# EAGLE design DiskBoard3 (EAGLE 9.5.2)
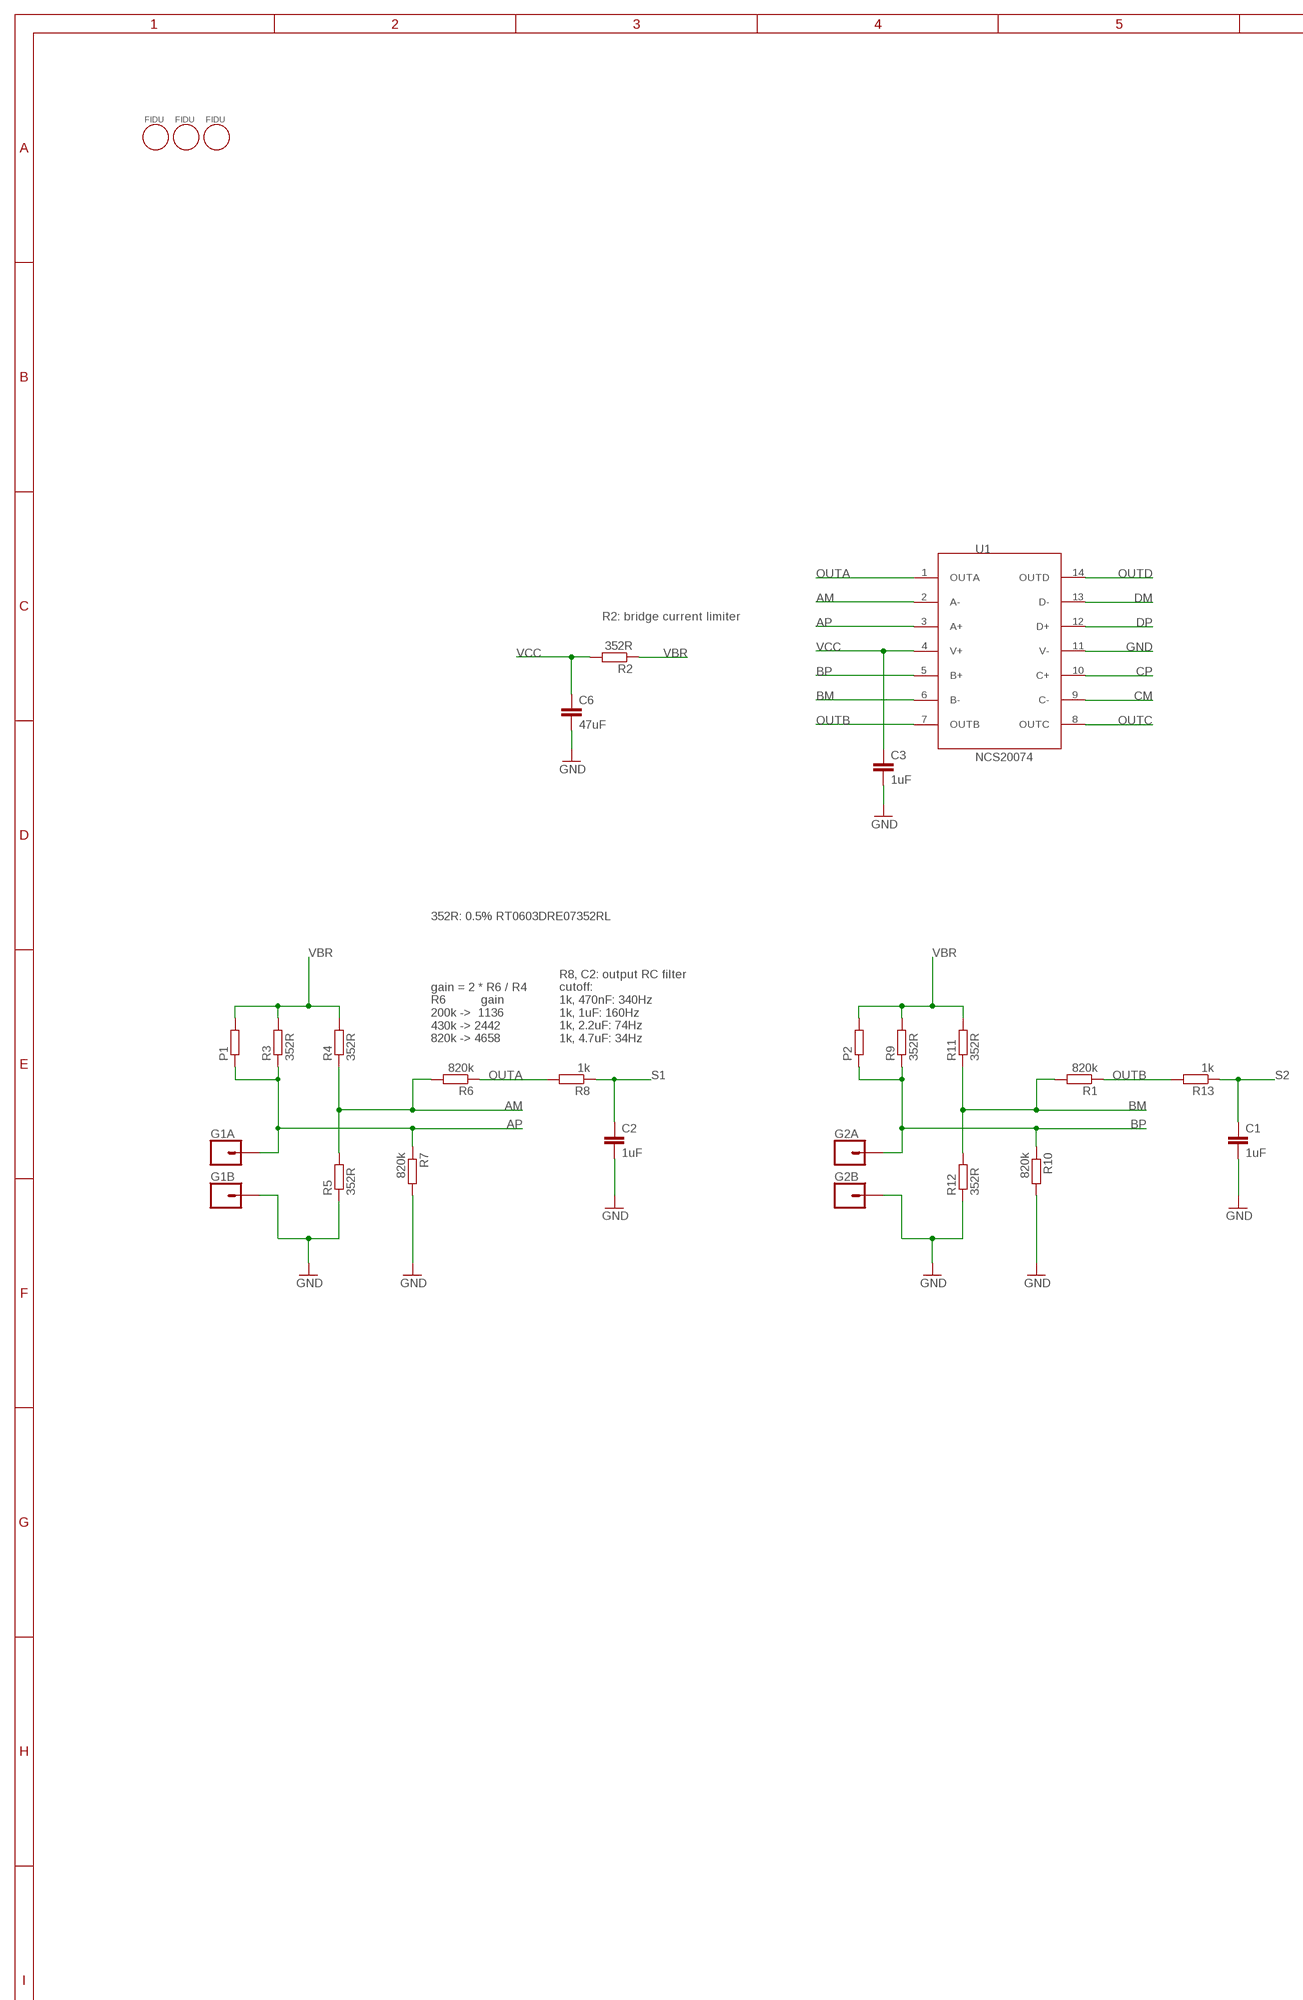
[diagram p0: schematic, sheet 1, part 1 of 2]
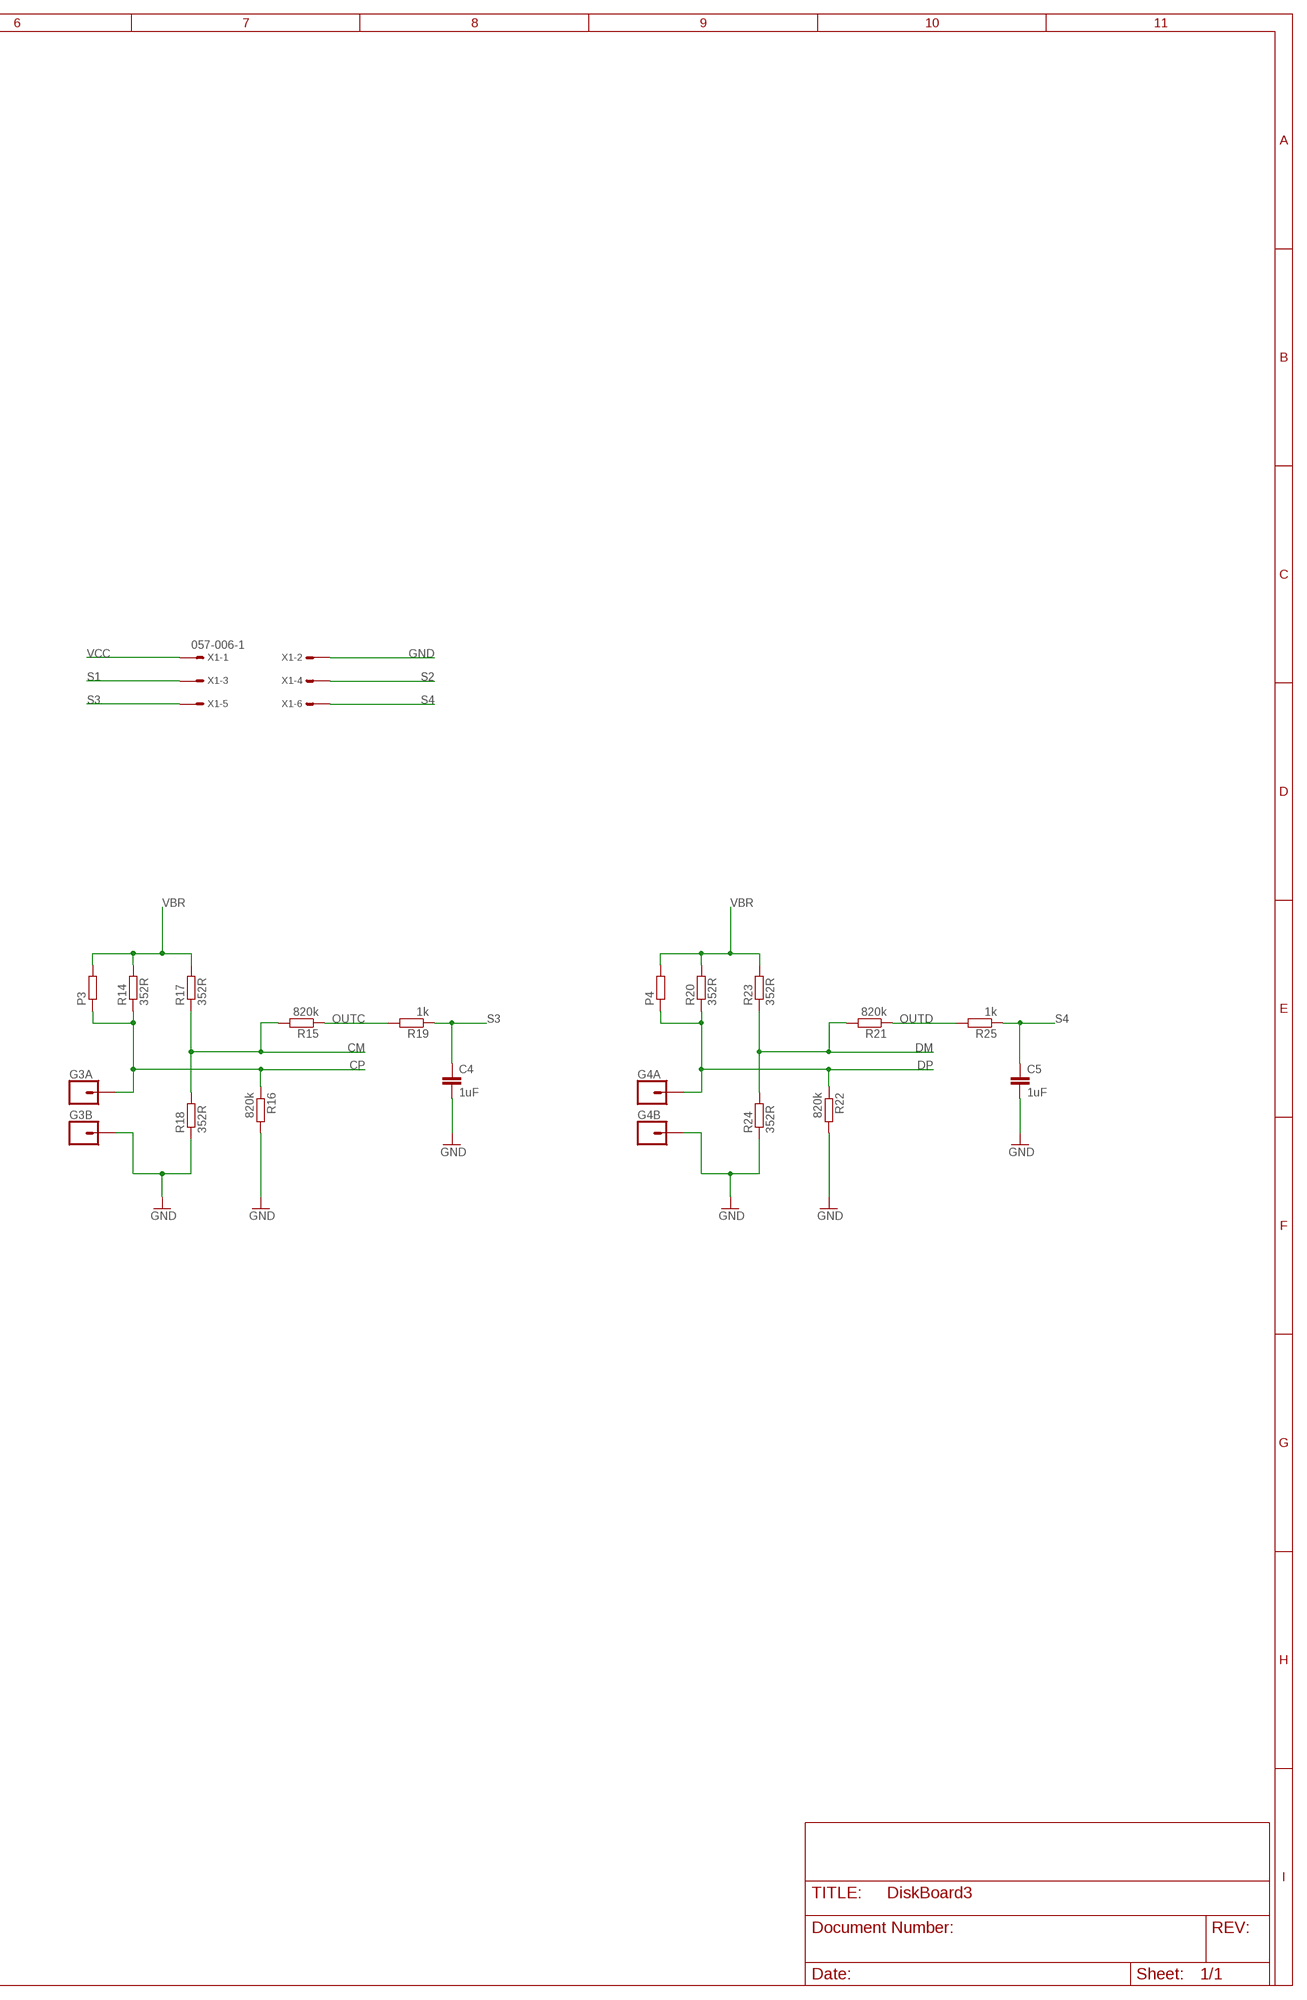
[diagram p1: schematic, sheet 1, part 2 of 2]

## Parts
C1  1uF  C-EUC0603  [C0603]
C2  1uF  C-EUC0603  [C0603]
C3  1uF  C-EUC0603  [C0603]
C4  1uF  C-EUC0603  [C0603]
C5  1uF  C-EUC0603  [C0603]
C6  47uF  C-EUC0603  [C0603]
G1A  THIN-CONNECTOR  [THIN-CONNECTOR]
G1B  THIN-CONNECTOR  [THIN-CONNECTOR]
G2A  THIN-CONNECTOR  [THIN-CONNECTOR]
G2B  THIN-CONNECTOR  [THIN-CONNECTOR]
G3A  THIN-CONNECTOR  [THIN-CONNECTOR]
G3B  THIN-CONNECTOR  [THIN-CONNECTOR]
G4A  THIN-CONNECTOR  [THIN-CONNECTOR]
G4B  THIN-CONNECTOR  [THIN-CONNECTOR]
P1  R-EU_0207/7  [0207/7]
P2  R-EU_0207/7  [0207/7]
P3  R-EU_0207/7  [0207/7]
P4  R-EU_0207/7  [0207/7]
R1  820k  R-EU_R0603  [R0603]
R2  352R  R-EU_R0603  [R0603]
R3  352R  R-EU_R0603  [R0603]
R4  352R  R-EU_R0603  [R0603]
R5  352R  R-EU_R0603  [R0603]
R6  820k  R-EU_R0603  [R0603]
R7  820k  R-EU_R0603  [R0603]
R8  1k  R-EU_R0603  [R0603]
R9  352R  R-EU_R0603  [R0603]
R10  820k  R-EU_R0603  [R0603]
R11  352R  R-EU_R0603  [R0603]
R12  352R  R-EU_R0603  [R0603]
R13  1k  R-EU_R0603  [R0603]
R14  352R  R-EU_R0603  [R0603]
R15  820k  R-EU_R0603  [R0603]
R16  820k  R-EU_R0603  [R0603]
R17  352R  R-EU_R0603  [R0603]
R18  352R  R-EU_R0603  [R0603]
R19  1k  R-EU_R0603  [R0603]
R20  352R  R-EU_R0603  [R0603]
R21  820k  R-EU_R0603  [R0603]
R22  820k  R-EU_R0603  [R0603]
R23  352R  R-EU_R0603  [R0603]
R24  352R  R-EU_R0603  [R0603]
R25  1k  R-EU_R0603  [R0603]
U1  NCS20074  [SOIC-14]
U$1  FIDUCIAL-3  [FIDUCIAL-3]
U$3  FIDUCIAL-3  [FIDUCIAL-3]
U$4  FIDUCIAL-3  [FIDUCIAL-3]
X1  057-006-1  [057-006-1]

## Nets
AM: R4.1 R5.2 R6.2 U1.2(A-)
AP: G1A.1 P1.1 R3.1 R7.1 U1.3(A+)
BM: R1.2 R11.1 R12.2 U1.6(B-)
BP: G2A.1 P2.1 R9.1 R10.1 U1.5(B+)
CM: R15.2 R17.1 R18.2 U1.9(C-)
CP: G3A.1 P3.1 R14.1 R16.1 U1.10(C+)
DM: R21.2 R23.1 R24.2 U1.13(D-)
DP: G4A.1 P4.1 R20.1 R22.1 U1.12(D+)
GND: C1.2 C2.2 C3.2 C4.2 C5.2 C6.2 G1B.1 G2B.1 G3B.1 G4B.1 R5.1 R7.2 R10.2 R12.1 R16.2 R18.1 R22.2 R24.1 U1.11(V-) X1.2
OUTA: R6.1 R8.2 U1.1(OUTA)
OUTB: R1.1 R13.2 U1.7(OUTB)
OUTC: R15.1 R19.2 U1.8(OUTC)
OUTD: R21.1 R25.2 U1.14(OUTD)
S1: C2.1 R8.1 X1.3
S2: C1.1 R13.1 X1.4
S3: C4.1 R19.1 X1.5
S4: C5.1 R25.1 X1.6
VBR: P1.2 P2.2 P3.2 P4.2 R2.1 R3.2 R4.2 R9.2 R11.2 R14.2 R17.2 R20.2 R23.2
VCC: C3.1 C6.1 R2.2 U1.4(V+) X1.1

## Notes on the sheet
- R2: bridge current limiter
- 352R: 0.5% RT0603DRE07352RL
- gain = 2 * R6 / R4
  R6          gain
  200k ->  1136
  430k -> 2442
  820k -> 4658
- R8, C2: output RC filter
  cutoff:
  1k, 470nF: 340Hz
  1k, 1uF: 160Hz
  1k, 2.2uF: 74Hz
  1k, 4.7uF: 34Hz

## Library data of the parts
C1-C6 = rcl:C-EU: CAPACITOR, European symbol; SPICEPREFIX: C
G1A G1B G2A G2B G3A G3B G4A G4B = nobo:THIN-CONNECTOR
P1-P4 R1-R25 = rcl:R-EU_: RESISTOR, European symbol; SPICEPREFIX: R
U1 = nobo:NCS20074: Operational Amplifier, Railto-Rail Output, 3 MHz BW https://hu.mouser.com/datasheet/2/308/NCS20071-D-470030.pdf
U$1 U$3 U$4 = nobo:FIDUCIAL-3
X1 = con-panduit:057-006-: CONNECTOR 6-pin series 057 contact pc board low profile headers; OC_FARNELL: unknown; OC_NEWARK: unknown

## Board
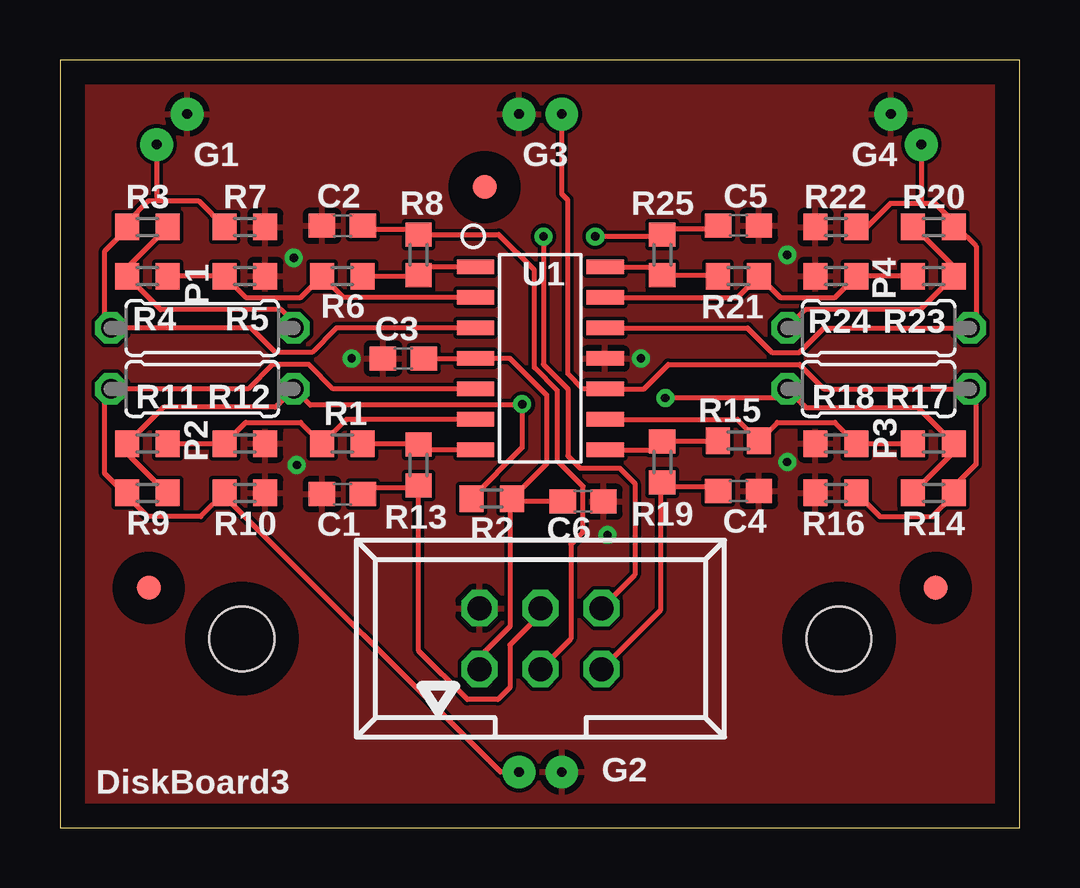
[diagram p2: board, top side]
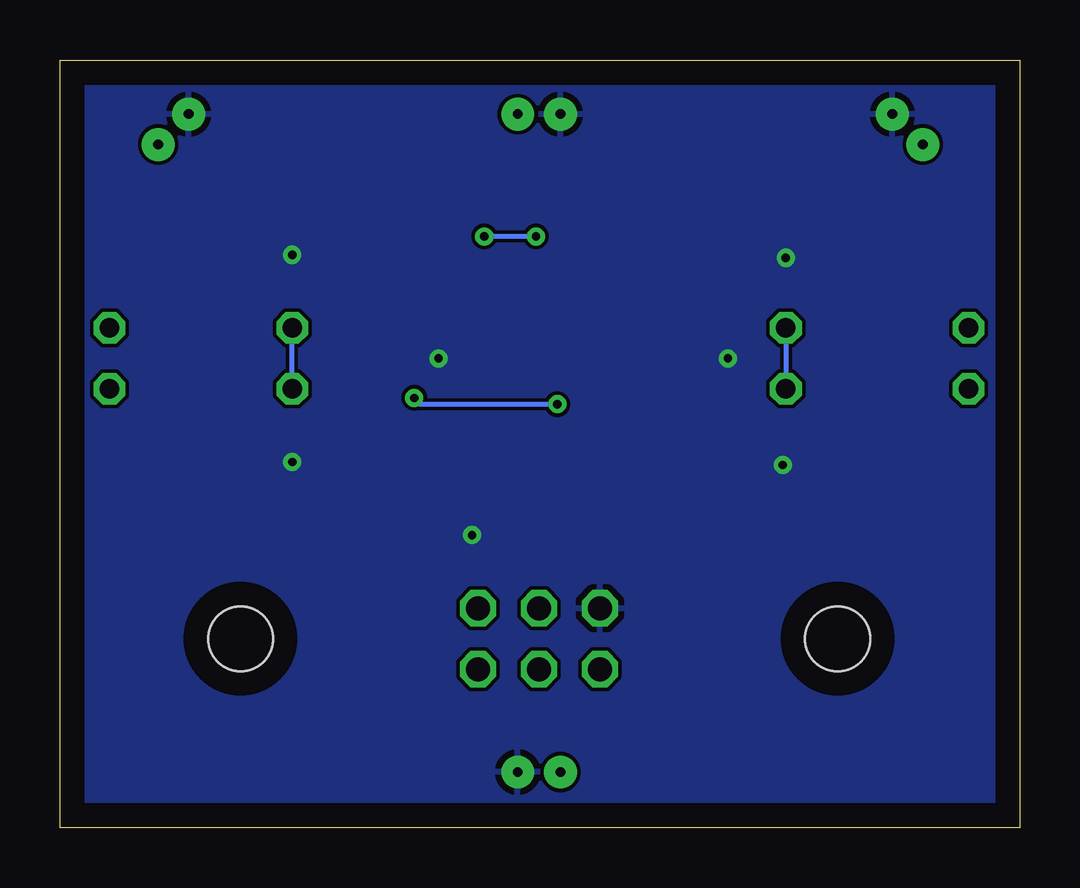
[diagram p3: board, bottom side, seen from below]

Size 40 x 32 mm. Coordinates in mm from the lower left corner, seen from the top.
Outline: 0,0 40,0 40,32 0,32 0,0
Copper layers (1*16): Top 0.035mm / dielectric 1.5mm / Bottom 0.035mm
Design rules "default": minimum track width 6mil, minimum drill 0.35mm, track to track 6mil, track to pad 6mil, pad to pad 6mil, via to via 6mil, smd to smd 6mil, copper to edge 40mil, drill to drill 6mil, minimum pad ring 10mil, minimum via ring 8mil, stop-mask expansion 4mil, vias tented up to drill 0mil, thermal gap 10mil
Holes 2.69 mm at 7.58,7.87 32.48,7.87

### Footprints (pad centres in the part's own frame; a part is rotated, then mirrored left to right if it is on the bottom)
C0603 = smd 1.1 x 1: 1 -0.85,0; 2 0.85,0
THIN-CONNECTOR = drill 0.406 pad 1.372: 1 0,0
0207/7 = drill 0.813 octagon: 1 -3.81,0; 2 3.81,0
R0603 = smd 1 x 1.1: 1 -0.85,0; 2 0.85,0
SOIC-14 = smd 0.6 x 1.55: 1 -3.81,-2.7; 2 -2.54,-2.7; 3 -1.27,-2.7; 4 0,-2.7; 5 1.27,-2.7; 6 2.54,-2.7; 7 3.81,-2.7; 8 3.81,2.7; 9 2.54,2.7; 10 1.27,2.7; 11 0,2.7; 12 -1.27,2.7; 13 -2.54,2.7; 14 -3.81,2.7
FIDUCIAL-3 = smd 1 x 1: 1 0,0
057-006-1 = drill 1 octagon: 1 -2.54,-1.27; 2 -2.54,1.27; 3 0,-1.27; 4 0,1.27; 5 2.54,-1.27; 6 2.54,1.27

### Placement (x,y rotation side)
C1  11.77,13.9 180 top
C2  11.77,25.09 180 top
C3  14.31,19.56 180 top
C4  28.28,14.02 0 top
C5  28.28,25.09 0 top
C6  21.81,13.59 0 top
G1A  4.03,28.48 0 top
G1B  5.3,29.75 0 top
G2A  19.14,2.31 0 top
G2B  20.92,2.31 0 top
G3A  20.92,29.75 0 top
G3B  19.14,29.75 0 top
G4A  35.9,28.48 0 top
G4B  34.63,29.75 0 top
P1  5.93,20.83 0 top
P2  5.93,18.29 0 top
P3  34.13,18.29 180 top
P4  34.13,20.83 180 top
R1  11.77,16 180 top
R2  18,13.72 0 top
R3  3.65,25.04 0 top
R4  3.65,22.99 180 top
R5  7.71,22.99 180 top
R6  11.77,22.99 180 top
R7  7.71,25.04 0 top
R8  14.95,23.88 270 top
R9  3.65,13.95 0 top
R10  7.71,13.95 0 top
R11  3.65,16 180 top
R12  7.71,16 180 top
R13  14.95,15.11 90 top
R14  36.41,13.95 180 top
R15  28.28,16.13 0 top
R16  32.35,13.95 180 top
R17  36.41,16 0 top
R18  32.35,16 0 top
R19  25.11,15.24 90 top
R20  36.41,25.04 180 top
R21  28.28,22.99 0 top
R22  32.35,25.04 180 top
R23  36.41,22.99 0 top
R24  32.35,22.99 0 top
R25  25.11,23.88 270 top
U1  20.03,19.56 270 top
U$1  17.7,26.7 0 top
U$3  3.7,10 0 top
U$4  36.5,10 0 top
X1  20.03,7.87 0 top

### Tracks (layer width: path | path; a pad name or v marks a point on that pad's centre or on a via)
AM
  Top 0.203: R4.1 R5.2 7.75,22.1 10.04,22.1 R6.2 11.81,22.1 U1.2
AP
  Top 0.203: U1.3 11.52,20.83 10.5,19.81 8.98,19.81 7.96,20.83 P1.1 1.87,21.08 1.87,24.04 2.8,24.96 R3.1 2.8,25.24 3.69,26.13 4.03,26.13 | R7.1 5.77,26.13 4.03,26.13 | G1A.1 4.03,26.13
BM
  Top 0.203: R11.1 R12.2 7.75,16.89 10.04,16.89 R1.2 11.94,17.02 U1.6
BP
  Top 0.203: U1.5 11.39,18.29 10.38,19.3 8.85,19.3 7.84,18.29 P2.1 1.87,18.03 1.87,14.75 2.67,13.95 | R9.1 2.67,13.95 | 2.67,13.95 3.66,12.96 5.87,12.96 R10.1 6.86,13.81 18.36,2.31 G2A.1
CM
  Top 0.203: U1.9 28.25,17.02 R15.2 29.9,16.89 32.31,16.89 R18.2 R17.1
CP
  Top 0.203: R16.1 34.19,12.96 36.37,12.96 37.26,13.85 R14.1 37.26,14.22 38.19,15.15 38.19,18.03 P3.1 31.84,18.29 30.82,19.3 25.36,19.3 24.35,18.29 U1.10 21.81,18.29 21.17,18.92 21.17,26.16 20.92,26.42 G3A.1
DM
  Top 0.203: R23.1 R24.2 32.31,22.1 30.02,22.1 R21.2 28.25,22.1 U1.13
DP
  Top 0.203: R22.1 33.65,25.04 34.63,26.03 35.9,26.03 | 35.9,26.03 36.47,26.03 37.26,25.24 R20.1 37.39,25.04 38.19,24.24 38.19,21.08 P4.1 31.84,20.83 30.82,19.81 29.68,19.81 28.66,20.83 U1.12 | G4A.1 35.9,26.03
GND  (via drill 0.35)
  other vias: 12.15,19.56 24.22,19.56 9.87,15.11 9.74,23.75 30.32,23.88 30.32,15.24 22.82,12.19
  pour Bottom: 0.28,39.38 44.58,39.38 50.04,33.92 50.04,0.03 44.55,-5.46 -1.57,-5.46 -4.56,-2.47 -4.56,34.54
  pour Top: 1,37.48 43.56,37.48 48.01,33.03 48.01,1.3 42.65,-4.06 -0.55,-4.06 -4.08,-0.54 -4.08,32.4
OUTA
  Top 0.203: R6.1 14.91,22.99 R8.2 15.29,23.37 U1.1
OUTB
  Top 0.203: R1.1 14.91,16 R13.2 15.16,15.75 U1.7
OUTC
  Top 0.203: R15.1 27.39,16.09 R19.2 24.98,15.96 24.85,15.96 24.63,15.75 U1.8
OUTD
  Top 0.203: U1.14 24.76,23.37 R25.2 27.39,23.03 R21.1
S1
  Top 0.203: C2.1 12.79,24.93 14.75,24.93 R8.1 18.29,24.73 19.77,23.24 19.77,19.18 20.73,18.22 20.73,15.3 21.81,14.22 21.81,12.32 21.3,11.81 21.3,7.87 X1.3
S2
  Top 0.203: X1.4 20.03,8.89 18.76,7.62 18.76,5.84 18.25,5.33 16.98,5.33 14.95,7.37 R13.1 14.85,14.16 12.89,14.16 C1.1
S3
  Top 0.203: X1.5 25.05,9.08 25.05,14.39 R19.1 25.31,14.19 27.27,14.19 C4.1
S4  (via drill 0.35)
  Top 0.203: v22.32,24.64 25.02,24.64 R25.1 25.34,24.95 27.3,24.95 C5.1 | X1.6 23.97,10.54 23.97,14.35 23.33,14.99 21.68,14.99 21.17,15.49 21.17,18.29 20.16,19.3 v20.16,24.64
  Bottom 0.203: v20.16,24.64 v22.32,24.64
VBR  (via drill 0.35)
  Top 0.203: R20.2 35.61,25.04 37.26,23.39 R23.2 35.87,21.59 31.08,21.59 P4.2 | R14.2 37.26,15.65 R17.2 35.76,17.51 31.1,17.51 P3.2 29.93,17.91 v25.24,17.91 | R3.2 2.8,23.34 R4.2 4.19,21.59 9.23,21.59 9.74,21.08 P1.2 | R9.2 4.45,13.95 2.8,15.6 R11.2 4.32,17.53 8.98,17.53 P2.2 10.43,17.61 19.22,17.61 v19.27,17.65 19.27,15.84 R2.1
  Bottom 0.203: P3.2 P4.2 | P1.2 P2.2 | v19.27,17.65 24.98,17.65 v25.24,17.91
VCC
  Top 0.203: C3.1 U1.4 18.76,19.56 20.28,18.03 20.28,15.15 R2.2 18.76,13.63 18.76,13.59 | X1.1 17.49,7.11 18.76,8.38 18.76,13.59 | C6.1 18.76,13.59

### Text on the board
tNames: G1 | G3 | G4 | G2 | DiskBoard3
